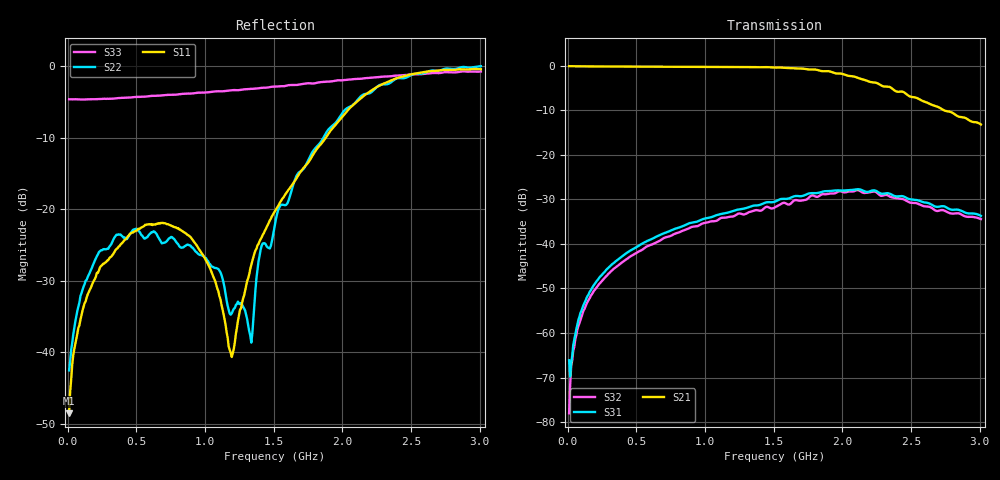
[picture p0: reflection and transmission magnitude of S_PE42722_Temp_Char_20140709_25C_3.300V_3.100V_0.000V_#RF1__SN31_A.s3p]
! Device ID: PE42722_Temp_Char_20140709
! Dir: c:\SVN\PSC 4Port_VNA Bench\CVI 2009\datafile\PE42722\PE42722_Temp_Char_20140709\25C\3p300000\#RF1
! Serial: 31
! Insertion: A
! Temp: 25C
! VDD: 3.300
! Control_Hi: 3.100
! Control_Lo: 0.000
! Logic State: #RF1
! ThroughPath: 2-1
! Port 1: RFC
! Port 2: RF1
! Port 3: RF2
! IDD: 1.151578e-04
! FILE NAME
! DATE 07/10/14  13:51
! CORRECTED  DATA
#  Hz  S  RI  R  75
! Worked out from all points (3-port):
!   401 points, 10 MHz to 3.01 GHz, reference 75 ohm
!   strongest paths, dB at 10 MHz, 760 MHz, 1.51 GHz, 2.26 GHz, 3.01 GHz:
!     S21: -0.1, -0.3, -0.5, -4.0, -13.2
!     S31: -66.1, -36.9, -30.5, -28.4, -33.7
!     S32: -78.0, -38.1, -31.8, -28.7, -34.5
!   lowest |S11| = -48.5 dB at 10 MHz (marker M1), VSWR 1.01, Z = 75.3 + j0.491 ohm
!   |S11| at or under -10 dB: start of sweep to 1.881 GHz
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1e7  0.00187 0.00326  0.9835 -0.0113  -0.000107 0.000122
     0.9843 -0.0112  0.00675 0.00324  3.05e-05 -0.000146
     0.000392 0.0003  -1.96e-05 -0.000124  -0.5861 0.00687
1e8  0.00769 0.0164  0.975 -0.1057  0.000237 0.00179
     0.9753 -0.106  0.0139 0.0219  0.000328 0.00151
     0.000238 0.00176  0.000316 0.00149  -0.5827 0.0452
3.25e8  0.0271 0.0393  0.9182 -0.3293  0.00152 0.00569
        0.9175 -0.3301  0.027 0.0528  0.00238 0.00446
        0.00154 0.00574  0.00238 0.00448  -0.5769 0.1306
8.8e8  0.0428 0.0498  0.5695 -0.7843  0.0108 0.0128
       0.5686 -0.7852  0.0261 0.0499  0.0142 0.00374
       0.0111 0.0128  0.0144 0.00368  -0.5799 0.2762
1.195e9  0.00766 -0.00525  0.2462 -0.9387  0.0199 0.0128
         0.2434 -0.9341  0.000628 0.0187  0.0197 -0.00615
         0.0195 0.0124  0.0192 -0.0061  -0.5795 0.3495
1.3375e9  -0.0155 -0.0379  0.0713 -0.9655  0.0246 0.011
          0.0693 -0.9611  -0.0106 -0.00501  0.0202 -0.0121
          0.0241 0.011  0.0199 -0.0116  -0.5745 0.3881
1.405e9  -0.0247 -0.0566  -0.0141 -0.9654  0.0269 0.00983
         -0.0178 -0.9563  -0.0457 -0.025  0.0191 -0.0153
         0.0258 0.00966  0.0186 -0.0144  -0.5737 0.4063
1.51e9  -0.0504 -0.083  -0.1566 -0.9496  0.0304 0.00693
        -0.1592 -0.935  -0.0671 -0.041  0.0178 -0.0202
        0.0288 0.00737  0.0176 -0.0187  -0.5707 0.4373
2.035e9  -0.4611 -0.1469  -0.7285 -0.3668  0.0328 -0.0234
         -0.6722 -0.3826  -0.4907 -0.1322  -0.0158 -0.0333
         0.0341 -0.0206  -0.0151 -0.0351  -0.5924 0.5402
3.01e9  -0.9413 0.1276  -0.1795 0.1083  -7.96e-05 -0.0204
        -0.175 0.1306  -0.9977 -0.00998  -0.0155 0.0125
        -0.00233 -0.0205  -0.0148 0.0118  -0.8923 0.2099
